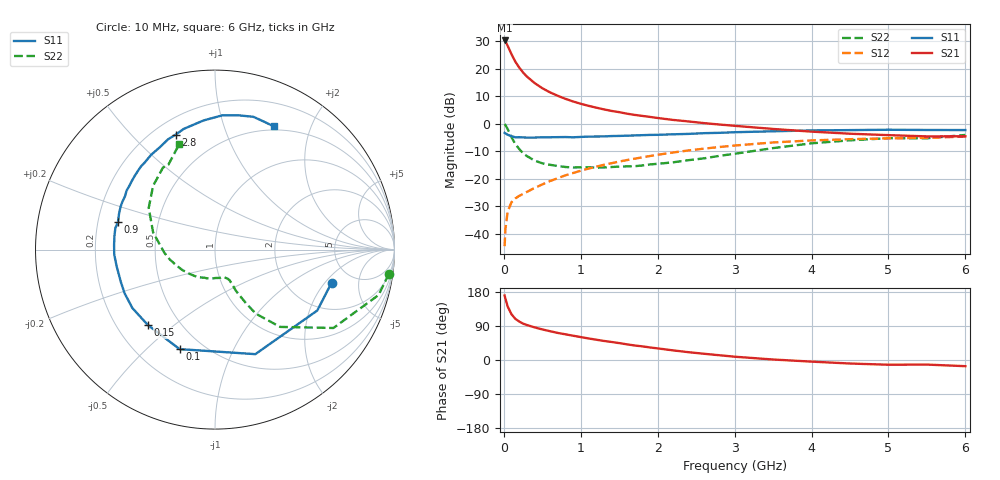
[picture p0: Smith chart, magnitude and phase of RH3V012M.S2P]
! SIEMENS Small Signal Semiconductors
! BFR106
! Si NPN RF Bipolar Junction Transistor in SOT23
! VCE = 3 V  IC = 12 mA
! Common Emitter S-Parameters:  August  1996
# GHz  S  MA  R  50
!  f  S11  S21  S12  S22
! GHz  MAG  ANG  MAG  ANG  MAG  ANG  MAG  ANG
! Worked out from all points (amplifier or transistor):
!   36 points, 10 MHz to 6 GHz, reference 50 ohm
!   highest |S21| = 30.2 dB at 10 MHz (marker M1)
!   |S21| within 3 dB of that: start of sweep to 67.05 MHz
!   unconditionally stable (mu >= 1): 448 MHz to 2.184 GHz; 5.165 GHz to end of sweep
!   at 250 MHz: K = 0.77, MSG = 22.1 dB, |S12| = -25.6 dB
!   at 1.4 GHz: K = 1.09, MAG = 7.7 dB, |S12| = -14.4 dB
!   at 6 GHz: K = 1.01, MAG = -0.6 dB, |S12| = -4.8 dB
!   S11 on the Smith chart (normalised r, x): 10 MHz: 3.46, -2.35; 100 MHz: 0.38, -0.64; 150 MHz: 0.33, -0.41; 900 MHz: 0.29, +0.13; 2.8 GHz: 0.29, +0.68; 6 GHz: 0.46, +1.48
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0.01  0.6752 -15.9  32.34 170.3  0.0059 82.5  0.9782 -7.9
0.02  0.6632 -30.8  31.38 162.3  0.0119 76.4  0.9461 -15.5
0.05  0.6244 -68.9  25.84 141.0  0.0253 61.6  0.7913 -33.5
0.1  0.5885 -109.6  18.11 120.5  0.0372 50.1  0.563 -49.9
0.15  0.5625 -131.8  13.26 108.5  0.0435 47.0  0.4234 -57.5
0.2  0.5638 -144.7  10.4 101.5  0.0484 47.8  0.3442 -60.0
0.25  0.5594 -154.1  8.453 96.0  0.0527 49.0  0.2885 -61.8
0.3  0.5547 -161.1  7.13 92.2  0.0571 51.7  0.2557 -63.1
0.4  0.556 -170.6  5.441 86.1  0.0675 54.9  0.2123 -63.8
0.5  0.5622 -177.3  4.38 80.7  0.0782 57.5  0.1892 -64.6
0.6  0.563 177.0  3.686 76.0  0.09 59.2  0.1776 -66.3
0.7  0.5653 172.1  3.194 71.5  0.1014 60.6  0.1692 -69.0
0.9  0.5621 164.1  2.516 64.1  0.126 61.5  0.1587 -74.3
1.1  0.578 155.5  2.1 56.9  0.1514 61.4  0.1593 -82.7
1.3  0.5831 149.3  1.808 50.3  0.1774 60.4  0.1588 -91.1
1.6  0.601 140.4  1.511 41.3  0.2167 58.2  0.1661 -106.1
2.2  0.637 123.9  1.163 25.4  0.2974 51.2  0.1971 -137.1
2.8  0.6772 108.8  0.96 12.6  0.3738 42.4  0.2581 -167.8
3.5  0.7226 95.0  0.797 1.3  0.4527 31.1  0.3575 164.6
4.5  0.7592 80.2  0.653 -9.3  0.5193 14.7  0.4953 134.1
5.5  0.7628 68.5  0.584 -12.1  0.55 4.2  0.5395 118.8
6  0.7606 64.6  0.586 -16.3  0.5785 -3.3  0.6197 108.8
